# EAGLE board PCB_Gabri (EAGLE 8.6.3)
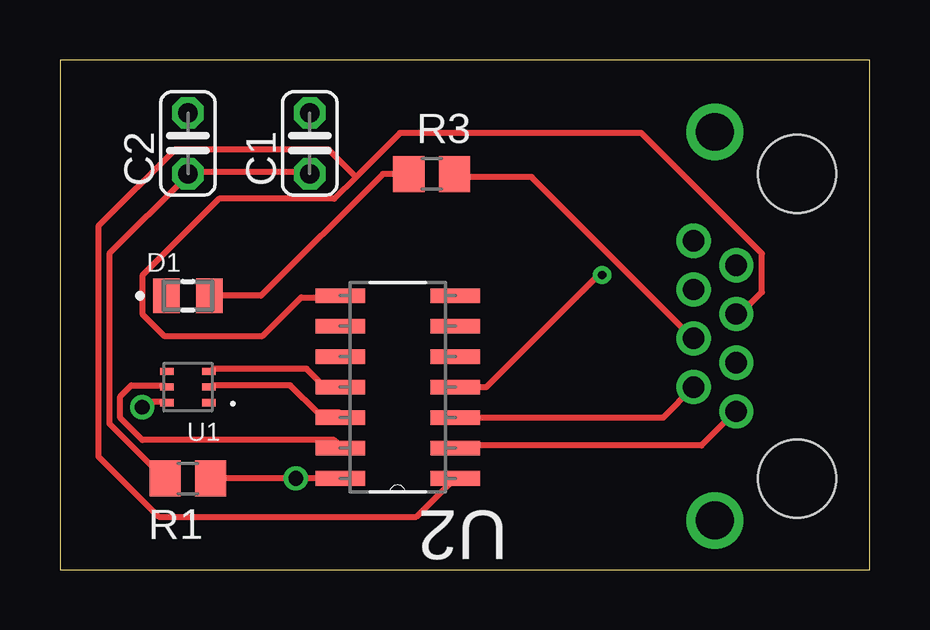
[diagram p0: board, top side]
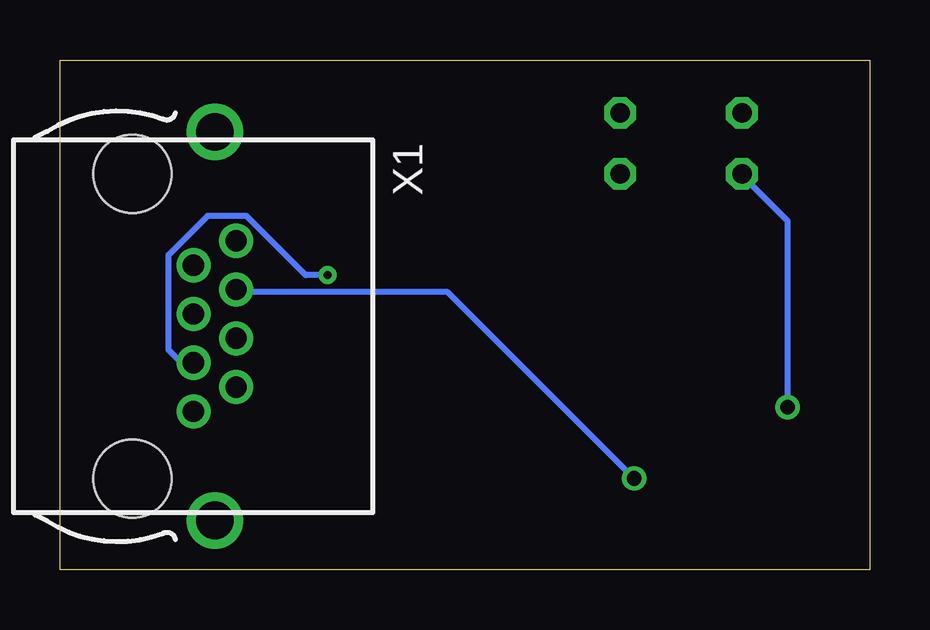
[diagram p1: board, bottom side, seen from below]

Size 33.76 x 21.26 mm. Coordinates in mm from the lower left corner, seen from the top.
Outline: 0,0 33.76,0 33.76,21.26 0,21.26 0,0
Copper layers (1*16): Top 0.035mm / dielectric 1.5mm / Bottom 0.035mm
Design rules "default": minimum track width 10mil, minimum drill 24mil, track to track 8mil, track to pad 8mil, pad to pad 8mil, via to via 8mil, smd to smd 8mil, copper to edge 40mil, drill to drill 8mil, minimum pad ring 10mil, minimum via ring 8mil, stop-mask expansion 4mil, vias tented up to drill 0mil, thermal gap 10mil
tRestrict: area 12.2,3.6 to 15.7,11.7; 8 lines

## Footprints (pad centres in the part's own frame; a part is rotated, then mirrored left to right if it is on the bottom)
C025-024X044 = drill 0.813 octagon: 1 -1.27,0; 2 1.27,0
LEDC2012X70N = smd 1.1 x 1.45: A 0.9,0; C -0.9,0
R0805 = smd 1.3 x 1.5: 1 -0.95,0; 2 0.95,0
VISHAY_VEML6030_2X2X0.87 = smd 0.55 x 0.3: 1 -0.875,0.65; 2 -0.875,0; 3 -0.875,-0.65; 4 0.875,-0.65; 5 0.875,0; 6 0.875,0.65
SOIC127P600X175-14N = smd 2.057 x 0.61: 1 -4.801,7.62; 2 -4.801,6.35; 3 -4.801,5.08; 4 -4.801,3.81; 5 -4.801,2.54; 6 -4.801,1.27; 7 -4.801,0; 8 0,0; 9 0,1.27; 10 0,2.54; 11 0,3.81; 12 0,5.08; 13 0,6.35; 14 0,7.62
0446200002 = drill 0.889 pad 1.422: 1 3.556,2.54; 2 2.54,4.318; 3 1.524,2.54; 4 0.508,4.318; 5 -0.508,2.54; 6 -1.524,4.318; 7 -2.54,2.54; 8 -3.556,4.318 | drill 1.575 pad 2.286: S@1 -8.103,3.429; S@2 8.103,3.429 | hole 3.251: 6.35,0; -6.35,0

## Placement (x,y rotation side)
C1  [C025-024X044]  10.41,17.78 90 top
C2  [C025-024X044]  5.33,17.78 90 top
D1  5988170107F  [LEDC2012X70N]  5.33,11.43 0 top
R1  [R0805]  5.33,3.81 180 top
R3  [R0805]  15.49,16.51 0 top
U1  VEML6030  [VISHAY_VEML6030_2X2X0.87]  5.33,7.62 180 top
U2  TXS0104ED  [SOIC127P600X175-14N]  11.68,11.43 180 top
X1  0446200002  [0446200002]  30.73,10.16 270 bottom

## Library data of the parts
C1 C2 R1 R3 = resistor
D1 = 5988170107F; AVAILABILITY: Unavailable; DESCRIPTION: LED GREEN CLEAR 0805 SMD; MF: Dialight; MP: 5988170107F; PACKAGE: 0805 Dialight; PRICE: None
U1 = VEML6030; AVAILABILITY: Unavailable; DESCRIPTION: VEML6030 Series 2 x 2 x 0.85 mm 50 mW I2C High Accuracy Ambient Light Sensor; MF: Vishay; MP: VEML6030; PACKAGE: SMD-6 Vishay; PRICE: None
U2 = TXS0104ED; AVAILABILITY: Unavailable; DESCRIPTION: 4-Bit Bidirectional Voltage-Level Shifter for Open-Drain and Push-Pull Applications 14-SOIC -40 to 85; MF: Texas Instruments; MP: TXS0104ED; PACKAGE: SOIC-14 Texas Instruments; PRICE: None
X1 = 0446200002; AVAILABILITY: Unavailable; DESCRIPTION: Conn RJ-45 RCP 8 POS 2.04mm Solder RA Thru-Hole 8 Terminal 1 Port Tray Cat 3; MF: Molex, LLC; MP: 0446200002; PACKAGE: None; PRICE: None

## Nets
GND: U1.1
N$1: C1.1 C2.1 R1.2 U1.6
N$3: U1.5 U2.13
N$4: U1.3 U2.11
N$5: U1.2 U2.12
N$6: D1.A R3.1
N$7: U2.2 X1.1
N$8: U2.3 X1.2
N$9: U2.4 X1.3
N$10: R1.1 U2.14 X1.6
N$12: R3.2 X1.4
N$17: U2.1 U2.8 X1.5

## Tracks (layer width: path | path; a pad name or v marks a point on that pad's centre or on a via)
N$1  (via drill 0.61)
  Top 0.254: v3.43,6.78 3.66,7.01 4.34,7.01 U1.6 | R1.2 4.34,3.81 2.06,6.1 2.06,13.18 5.26,16.38 C2.1 5.49,16.61 10.29,16.61 C1.1
  Bottom 0.254: v3.43,6.78 3.43,14.55 5.26,16.38 C2.1
N$3
  Top 0.254: U1.5 4.34,7.7 2.97,7.7 2.52,7.24 2.52,6.32 3.43,5.41 11.43,5.41 11.66,5.18 U2.13
N$4
  Top 0.254: U1.3 6.4,8.38 10.29,8.38 10.97,7.7 11.66,7.7 U2.11
N$5
  Top 0.254: U1.2 6.4,7.7 9.6,7.7 10.74,6.55 11.66,6.55 U2.12
N$6
  Top 0.254: R3.1 13.46,16.51 8.38,11.43 D1.A
N$7
  Top 0.254: U2.2 16.69,5.18 26.75,5.18 28.12,6.55 X1.1
N$8
  Top 0.254: U2.3 25.15,6.35 X1.2
N$9  (via drill 0.35)
  Top 0.254: U2.4 17.78,7.62 22.45,12.29 v22.61,12.29
  Bottom 0.254: X1.3 28.7,8.64 29.24,9.17 29.24,13.13 27.61,14.76 25.99,14.76 23.52,12.29 v22.61,12.29
N$10  (via drill 0.61)
  Top 0.254: U2.14 v9.83,3.81 R1.1
  Bottom 0.254: v9.83,3.81 17.6,11.58 26.29,11.58 X1.6
N$12
  Top 0.254: R3.2 16.46,16.38 19.66,16.38 26.29,9.75 X1.4
N$17
  Top 0.254: 12.34,16.38 14.17,18.21 24.23,18.21 29.26,13.18 29.26,11.58 28.35,10.67 X1.5 | 12.34,16.38 11.43,15.47 6.63,15.47 3.43,12.27 3.43,10.67 4.34,9.75 8.46,9.75 10.06,11.35 11.66,11.35 U2.8 | 12.34,16.38 11.2,17.53 4.8,17.53 1.6,14.33 1.6,4.72 4.12,2.21 14.86,2.21 16.46,3.81 U2.1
